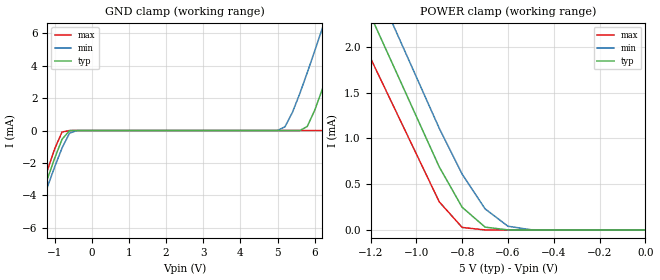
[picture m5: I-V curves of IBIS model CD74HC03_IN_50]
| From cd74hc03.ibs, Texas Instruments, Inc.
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|   CD74HC03 Input_IN_50
[Model]   CD74HC03_IN_50
Model_type  Input
Polarity   Inverting
Vinl = 1.8V
Vinh = 4.2V
| variable   typ   min   max
C_comp   1.930pf   1.534pf   2.323pf
[Temperature Range]   25   85   -40
[Voltage range]   5.0   4.5   6.0
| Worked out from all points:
|   GND clamp passes 1 mA (typ) near -0.88 V on its own axis
|   POWER clamp passes 1 mA (typ) near -0.96 V on its own axis
[GND Clamp]
|   Voltage   I(typ)   I(min)   I(max)
-5V       -29.88mA   -29.15mA   -30.41mA
-1.8V     -7.198mA   -7.497mA   -6.832mA
-1.6V     -5.79mA    -6.153mA   -5.366mA
-800mV    -540.3uA   -1.075mA   -91.15uA
-400mV    17.15nA    -602.9nA   15.16nA
5V        20.37nA    2.613uA    16.29nA
5.6V      901.8nA    2.281mA    16.59nA
5.8V      248.1uA    3.567mA    16.64nA
6.2V      2.512mA    6.27mA     16.77nA
6.8V      6.712mA    10.46mA    27.64uA
8V        15.4mA     18.97mA    6.064mA
10V       29.87mA    33.13mA    16.53mA
[POWER Clamp]
|   Voltage   I(typ)   I(min)   I(max)
-5V       23.32mA    24.13mA    21.77mA
-1.3V     2.896mA    3.356mA    2.401mA
-1.2V     2.344mA    2.795mA    1.877mA
-1.1V     1.793mA    2.234mA    1.354mA
-1V       1.241mA    1.672mA    830.6uA
-900mV    688.7uA    1.111mA    307.2uA
-800mV    248.1uA    609.8uA    27.64uA
-700mV    31.1uA     230.6uA    331.6nA
-600mV    901.8nA    40.89uA    19.28nA
-500mV    38.29nA    2.613uA    16.86nA
0V        20.37nA    20.99nA    16.77nA
